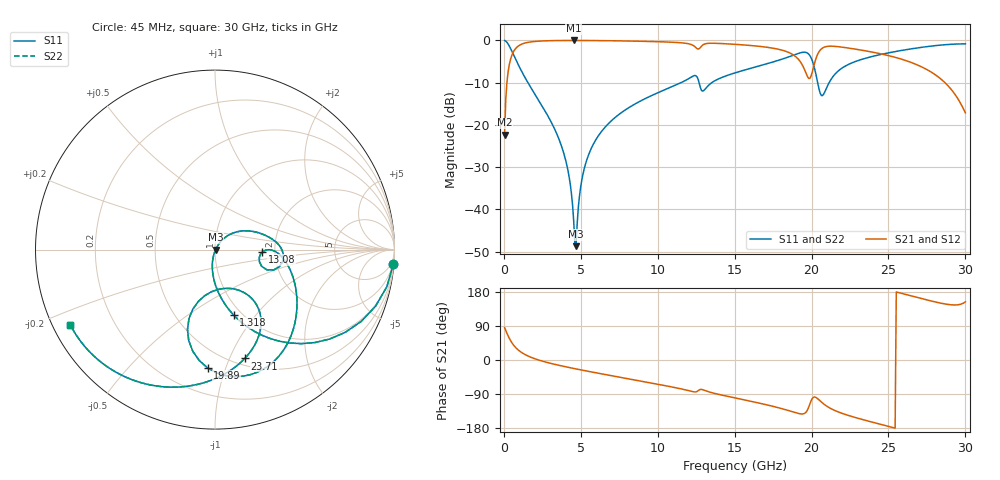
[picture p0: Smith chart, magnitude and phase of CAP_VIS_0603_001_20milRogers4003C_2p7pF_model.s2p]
! S-parameter model data by Modelithics Inc.  support@modelithics.com  813-866-6335  Tampa FL USA
! S-Parameter data specifications:
! Substrate: 20-mil Rogers 4003C, substrate thickness, H=0.508mm, Dielectric constant, Er=3.75
! PCB Mounting Pad Footprint: Pad width, PadW=0.90mm , Pad length, PadL=1.00mm , Pad gap, PadG (edge-to-edge)=1.00mm , Reference planes=3.0mm apart
! Created Wed Nov 18 13:20:56 2015
# hz S ma R 50
! 2 Port Network Data from SP1.SP block
! freq  magS11  angS11  magS21  angS21  magS12  angS12  magS22  angS22
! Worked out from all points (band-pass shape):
!   401 points, 45 MHz to 30 GHz, reference 50 ohm
!   highest |S21| = -0.03 dB at 4.538 GHz (marker M1); lowest = -22.3 dB at 45 MHz (marker M2)
!   |S21| within 3 dB of the highest: 574.6 MHz to 18.62 GHz (18.04 GHz wide, 188 % of centre); 20.43 GHz to 24.29 GHz (3.86 GHz wide, 17.3 % of centre)
!   lowest |S11| = -48.7 dB at 4.688 GHz (marker M3), VSWR 1.01, Z = 50.4 + j0.0469 ohm
!   |S11| at or under -10 dB: 1.56 GHz to 11.52 GHz (9.961 GHz wide, 152 % of centre); 12.69 GHz to 13.52 GHz (831.5 MHz wide, 6.35 % of centre); 20.39 GHz to 21.14 GHz (748.7 MHz wide, 3.61 % of centre)
!   |S22| runs from -48.7 to 0.0 dB; largest |S21 - S12| = 0
!   S11 on the Smith chart (normalised r, x): 45 MHz: 1, -25; 1.318 GHz: 0.92, -0.78; 13.08 GHz: 1.72, -0.05; 19.89 GHz: 0.37, -0.87; 23.71 GHz: 0.57, -1.14; 30 GHz: 0.05, -0.24
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4.5e7  0.997 -4.6  0.07677 85.4  0.07677 85.4  0.997 -4.6
4.194375e8  0.81 -38.0  0.5858 52.0  0.5858 52.0  0.81 -38.0
1.318088e9  0.3781 -74.2  0.9241 15.6  0.9241 15.6  0.3781 -74.2
3.714488e9  0.0582 -102.5  0.9952 -15.3  0.9952 -15.3  0.0582 -102.5
4.2387e9  0.0243 -102.8  0.9964 -19.8  0.9964 -19.8  0.0243 -102.8
4.53825e9  0.007217 -86.9  0.9965 -22.4  0.9965 -22.4  0.007217 -86.9
4.688025e9  0.003679 7.3  0.9964 -23.6  0.9964 -23.6  0.003679 7.3
5.062462e9  0.02219 54.9  0.996 -26.6  0.996 -26.6  0.02219 54.9
6.560212e9  0.09323 49.5  0.9912 -38.2  0.9912 -38.2  0.09323 49.5
1.007992e10  0.2433 24.0  0.9631 -64.6  0.9631 -64.6  0.2433 24.0
1.232655e10  0.3798 -3.1  0.865 -83.9  0.865 -83.9  0.3798 -3.1
1.307542e10  0.2646 -2.9  0.9086 -80.7  0.9086 -80.7  0.2646 -2.9
1.50225e10  0.4123 -11.7  0.8975 -100.0  0.8975 -100.0  0.4123 -11.7
1.86171e10  0.6472 -49.8  0.7053 -134.8  0.7053 -134.8  0.6472 -49.8
1.989019e10  0.6604 -93.6  0.3553 -116.0  0.3553 -116.0  0.6604 -93.6
2.003996e10  0.5801 -102.3  0.4179 -102.0  0.4179 -102.0  0.5801 -102.3
2.071395e10  0.2223 -76.6  0.8112 -113.6  0.8112 -113.6  0.2223 -76.6
2.176238e10  0.4389 -55.0  0.8404 -137.5  0.8404 -137.5  0.4389 -55.0
2.370945e10  0.6287 -74.7  0.74 -161.5  0.74 -161.5  0.6287 -74.7
2.505742e10  0.7146 -89.1  0.6562 -175.8  0.6562 -175.8  0.7146 -89.1
2.767849e10  0.8509 -119.8  0.4321 156.7  0.4321 156.7  0.8509 -119.8
3e10  0.9085 -152.6  0.1389 153.5  0.1389 153.5  0.9085 -152.6
